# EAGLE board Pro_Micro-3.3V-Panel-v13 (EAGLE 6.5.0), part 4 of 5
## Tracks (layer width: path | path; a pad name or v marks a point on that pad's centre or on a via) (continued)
N$120 (continued)
  Top 0.203: Y14.3 36.66,84.61 C123.1 35.82,86.19 33.86,86.19 33.48,86.56 33.48,87.13 32.43,88.18 31.7,88.18 31.24,88.64 31.24,88.89 30.89,89.25 30.89,90.16 30.4,90.65 30.4,91.22 30.78,91.6 31.15,91.6 31.33,91.78
N$121
  Top 0.203: C125.2 29.17,98.65 30.01,97.82 30.71,97.82 U28.6
N$122
  Top 0.203: X14.D-1 34.69,108.47 34.92,108.23 36.79,108.23 37,108.43 R84.2
N$123
  Top 0.203: X14.D+1 34.04,108.25 34.44,107.85 35.94,107.85 36.78,107 R83.2
N$124
  Top 0.203: F14.2 32.64,106.42 32.89,106.67 D42.2 31.98,107.99 31.98,109.12 31.75,109.35 31.5,109.35 29.84,111 27.94,111 27.43,111.51 27.05,111.51 26.83,111.73 SJ14.1
N$125
  Top 0.203: R82.2 D41.C
N$126
  Top 0.203: R81.2 D40.C
N$127
  Top 0.203: R85.1 47.75,106.92 LED15.A
N$128
  Top 0.203: Y15.1 50.6,81.53 51.82,82.74 51.82,84.8 C133.1 51.27,86.97 50.48,87.76 49.79,87.76 49.12,88.42 49.12,88.66 48.76,89.03 48.76,90.02 48.28,90.5 48.28,91.42 | 49.27,92.13 49.14,92 48.87,92 48.28,91.42 | 48.28,91.42
N$129
  Top 0.203: Y15.3 54.95,84.61 C132.1 54.11,86.19 52.14,86.19 51.77,86.56 51.77,87.13 50.72,88.18 49.98,88.18 49.53,88.64 49.53,88.89 49.17,89.25 49.17,90.16 48.69,90.65 48.69,91.22 49.06,91.6 49.44,91.6 49.62,91.78
N$130
  Top 0.203: C134.2 47.46,98.65 48.3,97.82 48.99,97.82 U30.6
N$131
  Top 0.203: X15.D-1 52.97,108.47 53.21,108.23 55.08,108.23 55.28,108.43 R90.2
N$132
  Top 0.203: X15.D+1 52.32,108.25 52.73,107.85 54.23,107.85 55.07,107 R89.2
N$133
  Top 0.203: F15.2 50.92,106.42 51.17,106.67 D45.2 50.27,107.99 50.27,109.12 50.04,109.35 49.78,109.35 48.13,111 46.23,111 45.72,111.51 45.34,111.51 45.12,111.73 SJ15.1
N$134
  Top 0.203: R88.2 D44.C
N$135
  Top 0.203: R87.2 D43.C
N$136
  Top 0.203: R91.1 66.04,106.92 LED16.A
N$137
  Top 0.203: Y16.1 68.89,81.53 70.1,82.74 70.1,84.8 C142.1 69.56,86.97 68.77,87.76 68.08,87.76 67.41,88.42 67.41,88.66 67.04,89.03 67.04,90.02 66.57,90.5 66.57,91.42 | 67.56,92.13 67.43,92 67.16,92 66.57,91.42 | 66.57,91.42
N$138
  Top 0.203: Y16.3 73.24,84.61 C141.1 72.4,86.19 70.43,86.19 70.06,86.56 70.06,87.13 69.01,88.18 68.27,88.18 67.82,88.64 67.82,88.89 67.46,89.25 67.46,90.16 66.97,90.65 66.97,91.22 67.35,91.6 67.73,91.6 67.9,91.78
N$139
  Top 0.203: C143.2 65.75,98.65 66.58,97.82 67.28,97.82 U32.6
N$140
  Top 0.203: X16.D-1 71.26,108.47 71.5,108.23 73.37,108.23 73.57,108.43 R96.2
N$141
  Top 0.203: X16.D+1 70.61,108.25 71.02,107.85 72.52,107.85 73.36,107 R95.2
N$142
  Top 0.203: F16.2 69.21,106.42 69.46,106.67 D48.2 68.56,107.99 68.56,109.12 68.33,109.35 68.07,109.35 66.42,111 64.52,111 64.01,111.51 63.63,111.51 63.4,111.73 SJ16.1
N$143
  Top 0.203: R94.2 D47.C
N$144
  Top 0.203: R93.2 D46.C
N$145
  Top 0.203: R97.1 84.33,106.92 LED17.A
N$146
  Top 0.203: Y17.1 87.18,81.53 88.39,82.74 88.39,84.8 C151.1 87.84,86.97 87.06,87.76 86.36,87.76 85.7,88.42 85.7,88.66 85.33,89.03 85.33,90.02 84.86,90.5 84.86,91.42 | 85.84,92.13 85.72,92 85.45,92 84.86,91.42 | 84.86,91.42
N$147
  Top 0.203: Y17.3 91.53,84.61 C150.1 90.69,86.19 88.72,86.19 88.35,86.56 88.35,87.13 87.3,88.18 86.56,88.18 86.11,88.64 86.11,88.89 85.75,89.25 85.75,90.16 85.26,90.65 85.26,91.22 85.64,91.6 86.02,91.6 86.19,91.78
N$148
  Top 0.203: C152.2 84.04,98.65 84.87,97.82 85.57,97.82 U34.6
N$149
  Top 0.203: X17.D-1 89.55,108.47 89.79,108.23 91.66,108.23 91.86,108.43 R102.2
N$150
  Top 0.203: X17.D+1 88.9,108.25 89.31,107.85 90.81,107.85 91.65,107 R101.2
N$151
  Top 0.203: F17.2 87.5,106.42 87.75,106.67 D51.2 86.84,107.99 86.84,109.12 86.61,109.35 86.36,109.35 84.71,111 82.8,111 82.3,111.51 81.92,111.51 81.69,111.73 SJ17.1
N$152
  Top 0.203: R100.2 D50.C
N$153
  Top 0.203: R99.2 D49.C
N$154
  Top 0.203: R103.1 102.61,106.92 LED18.A
N$155
  Top 0.203: Y18.1 105.47,81.53 106.68,82.74 106.68,84.8 C160.1 106.13,86.97 105.35,87.76 104.65,87.76 103.99,88.42 103.99,88.66 103.62,89.03 103.62,90.02 103.15,90.5 103.15,91.42 | 104.13,92.13 104.01,92 103.73,92 103.15,91.42 | 103.15,91.42
N$156
  Top 0.203: Y18.3 109.82,84.61 C159.1 108.97,86.19 107.01,86.19 106.63,86.56 106.63,87.13 105.58,88.18 104.85,88.18 104.39,88.64 104.39,88.89 104.04,89.25 104.04,90.16 103.55,90.65 103.55,91.22 103.93,91.6 104.3,91.6 104.48,91.78
N$157
  Top 0.203: C161.2 102.32,98.65 103.16,97.82 103.86,97.82 U36.6
N$158
  Top 0.203: X18.D-1 107.84,108.47 108.08,108.23 109.94,108.23 110.15,108.43 R108.2
N$159
  Top 0.203: X18.D+1 107.19,108.25 107.59,107.85 109.09,107.85 109.94,107 R107.2
N$160
  Top 0.203: F18.2 105.79,106.42 106.04,106.67 D54.2 105.13,107.99 105.13,109.12 104.9,109.35 104.65,109.35 103,111 101.09,111 100.58,111.51 100.2,111.51 99.98,111.73 SJ18.1
N$161
  Top 0.203: R106.2 D53.C
N$162
  Top 0.203: R105.2 D52.C
RAW  (via drill 0.25)
  Top 0.203: 16.36,29.72 16.36,28.07 16.63,27.8 17.26,27.8 U2.1 | D2.1 16.23,33.43 | 16.23,33.43 15.19,34.47 v14.8,34.47 | C19.A 19.18,29.66 U2.3 17.24,29.72 16.36,29.72 | 16.36,29.72 16.36,30.59 16.22,30.74 16.22,33.42 16.23,33.43
  Bottom 0.203: JP6.1 23.37,36.58 21.34,38.61 16,38.61 14.8,37.4 v14.8,34.47
RAW1  (via drill 0.25)
  Top 0.203: 34.65,29.72 34.65,28.07 34.92,27.8 35.54,27.8 U1.1 | D6.1 34.52,33.43 | 34.52,33.43 33.48,34.47 v33.08,34.47 | C12.A 37.47,29.66 U1.3 35.53,29.72 34.65,29.72 | 34.65,29.72 34.65,30.59 34.51,30.74 34.51,33.42 34.52,33.43
  Bottom 0.203: JP3.1 41.66,36.58 39.62,38.61 34.29,38.61 33.08,37.4 v33.08,34.47
RAW2  (via drill 0.25)
  Top 0.203: 52.94,29.72 52.94,28.07 53.21,27.8 53.83,27.8 U5.1 | D9.1 52.81,33.43 | 52.81,33.43 51.77,34.47 v51.37,34.47 | C23.A 55.76,29.66 U5.3 53.81,29.72 52.94,29.72 | 52.94,29.72 52.94,30.59 52.8,30.74 52.8,33.42 52.81,33.43
  Bottom 0.203: JP9.1 59.94,36.58 57.91,38.61 52.58,38.61 51.37,37.4 v51.37,34.47
RAW3  (via drill 0.25)
  Top 0.203: 71.23,29.72 71.23,28.07 71.5,27.8 72.12,27.8 U7.1 | D12.1 71.09,33.43 | 71.09,33.43 70.05,34.47 v69.66,34.47 | C32.A 74.05,29.66 U7.3 72.1,29.72 71.23,29.72 | 71.23,29.72 71.23,30.59 71.08,30.74 71.08,33.42 71.09,33.43
  Bottom 0.203: JP13.1 78.23,36.58 76.2,38.61 70.87,38.61 69.66,37.4 v69.66,34.47
RAW4  (via drill 0.25)
  Top 0.203: 89.52,29.72 89.52,28.07 89.79,27.8 90.41,27.8 U9.1 | D15.1 89.38,33.43 | 89.38,33.43 88.34,34.47 v87.95,34.47 | C41.A 92.33,29.66 U9.3 90.39,29.72 89.52,29.72 | 89.52,29.72 89.52,30.59 89.37,30.74 89.37,33.42 89.38,33.43
  Bottom 0.203: JP17.1 96.52,36.58 94.49,38.61 89.15,38.61 87.95,37.4 v87.95,34.47
RAW5  (via drill 0.25)
  Top 0.203: 107.81,29.72 107.81,28.07 108.07,27.8 108.7,27.8 U11.1 | D18.1 107.67,33.43 | 107.67,33.43 106.63,34.47 v106.24,34.47 | C50.A 110.62,29.66 U11.3 108.68,29.72 107.81,29.72 | 107.81,29.72 107.81,30.59 107.66,30.74 107.66,33.42 107.67,33.43
  Bottom 0.203: JP21.1 114.81,36.58 112.78,38.61 107.44,38.61 106.24,37.4 v106.24,34.47
RAW6  (via drill 0.25)
  Top 0.203: 16.36,66.55 16.36,64.9 16.63,64.63 17.26,64.63 U13.1 | D21.1 16.23,70.26 | 16.23,70.26 15.19,71.3 v14.8,71.3 | C59.A 19.18,66.49 U13.3 17.24,66.55 16.36,66.55 | 16.36,66.55 16.36,67.42 16.22,67.57 16.22,70.25 16.23,70.26
  Bottom 0.203: JP25.1 23.37,73.41 21.34,75.44 16,75.44 14.8,74.23 v14.8,71.3
RAW7  (via drill 0.25)
  Top 0.203: 34.65,66.55 34.65,64.9 34.92,64.63 35.54,64.63 U15.1 | D24.1 34.52,70.26 | 34.52,70.26 33.48,71.3 v33.08,71.3 | C68.A 37.47,66.49 U15.3 35.53,66.55 34.65,66.55 | 34.65,66.55 34.65,67.42 34.51,67.57 34.51,70.25 34.52,70.26
  Bottom 0.203: JP29.1 41.66,73.41 39.62,75.44 34.29,75.44 33.08,74.23 v33.08,71.3
RAW8  (via drill 0.25)
  Top 0.203: 52.94,66.55 52.94,64.9 53.21,64.63 53.83,64.63 U17.1 | D27.1 52.81,70.26 | 52.81,70.26 51.77,71.3 v51.37,71.3 | C77.A 55.76,66.49 U17.3 53.81,66.55 52.94,66.55 | 52.94,66.55 52.94,67.42 52.8,67.57 52.8,70.25 52.81,70.26
  Bottom 0.203: JP33.1 59.94,73.41 57.91,75.44 52.58,75.44 51.37,74.23 v51.37,71.3
RAW9  (via drill 0.25)
  Top 0.203: 71.23,66.55 71.23,64.9 71.5,64.63 72.12,64.63 U19.1 | D30.1 71.09,70.26 | 71.09,70.26 70.05,71.3 v69.66,71.3 | C86.A 74.05,66.49 U19.3 72.1,66.55 71.23,66.55 | 71.23,66.55 71.23,67.42 71.08,67.57 71.08,70.25 71.09,70.26
  Bottom 0.203: JP37.1 78.23,73.41 76.2,75.44 70.87,75.44 69.66,74.23 v69.66,71.3
RAW10  (via drill 0.25)
  Top 0.203: 89.52,66.55 89.52,64.9 89.79,64.63 90.41,64.63 U21.1 | D33.1 89.38,70.26 | 89.38,70.26 88.34,71.3 v87.95,71.3 | C95.A 92.33,66.49 U21.3 90.39,66.55 89.52,66.55 | 89.52,66.55 89.52,67.42 89.37,67.57 89.37,70.25 89.38,70.26
  Bottom 0.203: JP41.1 96.52,73.41 94.49,75.44 89.15,75.44 87.95,74.23 v87.95,71.3
RAW11  (via drill 0.25)
  Top 0.203: 107.81,66.55 107.81,64.9 108.07,64.63 108.7,64.63 U23.1 | D36.1 107.67,70.26 | 107.67,70.26 106.63,71.3 v106.24,71.3 | C104.A 110.62,66.49 U23.3 108.68,66.55 107.81,66.55 | 107.81,66.55 107.81,67.42 107.66,67.57 107.66,70.25 107.67,70.26
  Bottom 0.203: JP45.1 114.81,73.41 112.78,75.44 107.44,75.44 106.24,74.23 v106.24,71.3
RAW12  (via drill 0.25)
  Top 0.203: 16.36,103.38 16.36,101.73 16.63,101.46 17.26,101.46 U25.1 | D39.1 16.23,107.09 | 16.23,107.09 15.19,108.13 v14.8,108.13 | C113.A 19.18,103.32 U25.3 17.24,103.38 16.36,103.38 | 16.36,103.38 16.36,104.25 16.22,104.4 16.22,107.08 16.23,107.09
  Bottom 0.203: JP49.1 23.37,110.24 21.34,112.27 16,112.27 14.8,111.06 v14.8,108.13
RAW13  (via drill 0.25)
  Top 0.203: 34.65,103.38 34.65,101.73 34.92,101.46 35.54,101.46 U27.1 | D42.1 34.52,107.09 | 34.52,107.09 33.48,108.13 v33.08,108.13 | C122.A 37.47,103.32 U27.3 35.53,103.38 34.65,103.38 | 34.65,103.38 34.65,104.25 34.51,104.4 34.51,107.08 34.52,107.09
  Bottom 0.203: JP53.1 41.66,110.24 39.62,112.27 34.29,112.27 33.08,111.06 v33.08,108.13
RAW14  (via drill 0.25)
  Top 0.203: 52.94,103.38 52.94,101.73 53.21,101.46 53.83,101.46 U29.1 | D45.1 52.81,107.09 | 52.81,107.09 51.77,108.13 v51.37,108.13 | C131.A 55.76,103.32 U29.3 53.81,103.38 52.94,103.38 | 52.94,103.38 52.94,104.25 52.8,104.4 52.8,107.08 52.81,107.09
  Bottom 0.203: JP57.1 59.94,110.24 57.91,112.27 52.58,112.27 51.37,111.06 v51.37,108.13
RAW15  (via drill 0.25)
  Top 0.203: 71.23,103.38 71.23,101.73 71.5,101.46 72.12,101.46 U31.1 | D48.1 71.09,107.09 | 71.09,107.09 70.05,108.13 v69.66,108.13 | C140.A 74.05,103.32 U31.3 72.1,103.38 71.23,103.38 | 71.23,103.38 71.23,104.25 71.08,104.4 71.08,107.08 71.09,107.09
  Bottom 0.203: JP61.1 78.23,110.24 76.2,112.27 70.87,112.27 69.66,111.06 v69.66,108.13
RAW16  (via drill 0.25)
  Top 0.203: 89.52,103.38 89.52,101.73 89.79,101.46 90.41,101.46 U33.1 | D51.1 89.38,107.09 | 89.38,107.09 88.34,108.13 v87.95,108.13 | C149.A 92.33,103.32 U33.3 90.39,103.38 89.52,103.38 | 89.52,103.38 89.52,104.25 89.37,104.4 89.37,107.08 89.38,107.09
  Bottom 0.203: JP65.1 96.52,110.24 94.49,112.27 89.15,112.27 87.95,111.06 v87.95,108.13
RAW17  (via drill 0.25)
  Top 0.203: 107.81,103.38 107.81,101.73 108.07,101.46 108.7,101.46 U35.1 | D54.1 107.67,107.09 | 107.67,107.09 106.63,108.13 v106.24,108.13 | C158.A 110.62,103.32 U35.3 108.68,103.38 107.81,103.38 | 107.81,103.38 107.81,104.25 107.66,104.4 107.66,107.08 107.67,107.09
  Bottom 0.203: JP69.1 114.81,110.24 112.78,112.27 107.44,112.27 106.24,111.06 v106.24,108.13
RESET  (via drill 0.25)
  Top 0.203: 11.65,19.52 11.57,19.44 11.57,19.43 11.42,19.28 11.2,19.28 10.69,19.79 10.69,20.34 10.92,20.57 10.92,21.08 9.4,22.61 9.4,31.47 8.84,32.03 8.84,32.45 9.4,33.01 9.4,35.18 v10.29,36.07 11.09,35.27 R2.1
  Bottom 0.203: JP6.3 22.1,32.26 22.1,34.04 22.48,34.42 22.48,35.18 22.1,35.56 22.1,37.08 21.01,38.18 18.16,38.18 16.79,36.8 16.79,34.29 15.8,33.3 13.06,33.3 v10.29,36.07
RESET1  (via drill 0.25)
  Top 0.203: 29.93,19.52 29.86,19.44 29.86,19.43 29.71,19.28 29.49,19.28 28.98,19.79 28.98,20.34 29.21,20.57 29.21,21.08 27.69,22.61 27.69,31.47 27.12,32.03 27.12,32.45 27.69,33.01 27.69,35.18 v28.57,36.07 29.38,35.27 R3.1
  Bottom 0.203: JP3.3 40.39,32.26 40.39,34.04 40.77,34.42 40.77,35.18 40.39,35.56 40.39,37.08 39.29,38.18 36.45,38.18 35.08,36.8 35.08,34.29 34.09,33.3 31.34,33.3 v28.57,36.07
RESET2  (via drill 0.25)
  Top 0.203: 48.22,19.52 48.15,19.44 48.15,19.43 48,19.28 47.78,19.28 47.27,19.79 47.27,20.34 47.5,20.57 47.5,21.08 45.97,22.61 45.97,31.47 45.41,32.03 45.41,32.45 45.97,33.01 45.97,35.18 v46.86,36.07 47.66,35.27 R14.1
  Bottom 0.203: JP9.3 58.67,32.26 58.67,34.04 59.05,34.42 59.05,35.18 58.67,35.56 58.67,37.08 57.58,38.18 54.74,38.18 53.37,36.8 53.37,34.29 52.38,33.3 49.63,33.3 v46.86,36.07
RESET3  (via drill 0.25)
  Top 0.203: 66.51,19.52 66.44,19.44 66.44,19.43 66.28,19.28 66.06,19.28 65.56,19.79 65.56,20.34 65.79,20.57 65.79,21.08 64.26,22.61 64.26,31.47 63.7,32.03 63.7,32.45 64.26,33.01 64.26,35.18 v65.15,36.07 65.95,35.27 R20.1
  Bottom 0.203: JP13.3 76.96,32.26 76.96,34.04 77.34,34.42 77.34,35.18 76.96,35.56 76.96,37.08 75.87,38.18 73.03,38.18 71.65,36.8 71.65,34.29 70.66,33.3 67.92,33.3 v65.15,36.07
RESET4  (via drill 0.25)
  Top 0.203: 84.8,19.52 84.72,19.44 84.72,19.43 84.57,19.28 84.35,19.28 83.84,19.79 83.84,20.34 84.07,20.57 84.07,21.08 82.55,22.61 82.55,31.47 81.99,32.03 81.99,32.45 82.55,33.01 82.55,35.18 v83.44,36.07 84.24,35.27 R26.1
  Bottom 0.203: JP17.3 95.25,32.26 95.25,34.04 95.63,34.42 95.63,35.18 95.25,35.56 95.25,37.08 94.16,38.18 91.31,38.18 89.94,36.8 89.94,34.29 88.95,33.3 86.21,33.3 v83.44,36.07
RESET5  (via drill 0.25)
  Top 0.203: 103.09,19.52 103.01,19.44 103.01,19.43 102.86,19.28 102.64,19.28 102.13,19.79 102.13,20.34 102.36,20.57 102.36,21.08 100.84,22.61 100.84,31.47 100.28,32.03 100.28,32.45 100.84,33.01 100.84,35.18 v101.73,36.07 102.53,35.27 R32.1
  Bottom 0.203: JP21.3 113.54,32.26 113.54,34.04 113.92,34.42 113.92,35.18 113.54,35.56 113.54,37.08 112.45,38.18 109.6,38.18 108.23,36.8 108.23,34.29 107.24,33.3 104.5,33.3 v101.73,36.07
RESET6  (via drill 0.25)
  Top 0.203: 11.65,56.34 11.57,56.27 11.57,56.26 11.42,56.11 11.2,56.11 10.69,56.62 10.69,57.17 10.92,57.4 10.92,57.91 9.4,59.44 9.4,68.3 8.84,68.86 8.84,69.28 9.4,69.84 9.4,72.01 v10.29,72.9 11.09,72.1 R38.1
  Bottom 0.203: JP25.3 22.1,69.09 22.1,70.87 22.48,71.25 22.48,72.01 22.1,72.39 22.1,73.91 21.01,75.01 18.16,75.01 16.79,73.64 16.79,71.12 15.8,70.13 13.06,70.13 v10.29,72.9
RESET7  (via drill 0.25)
  Top 0.203: 29.93,56.34 29.86,56.27 29.86,56.26 29.71,56.11 29.49,56.11 28.98,56.62 28.98,57.17 29.21,57.4 29.21,57.91 27.69,59.44 27.69,68.3 27.12,68.86 27.12,69.28 27.69,69.84 27.69,72.01 v28.57,72.9 29.38,72.1 R44.1
  Bottom 0.203: JP29.3 40.39,69.09 40.39,70.87 40.77,71.25 40.77,72.01 40.39,72.39 40.39,73.91 39.29,75.01 36.45,75.01 35.08,73.64 35.08,71.12 34.09,70.13 31.34,70.13 v28.57,72.9
RESET8  (via drill 0.25)
  Top 0.203: 48.22,56.34 48.15,56.27 48.15,56.26 48,56.11 47.78,56.11 47.27,56.62 47.27,57.17 47.5,57.4 47.5,57.91 45.97,59.44 45.97,68.3 45.41,68.86 45.41,69.28 45.97,69.84 45.97,72.01 v46.86,72.9 47.66,72.1 R50.1
  Bottom 0.203: JP33.3 58.67,69.09 58.67,70.87 59.05,71.25 59.05,72.01 58.67,72.39 58.67,73.91 57.58,75.01 54.74,75.01 53.37,73.64 53.37,71.12 52.38,70.13 49.63,70.13 v46.86,72.9
RESET9  (via drill 0.25)
  Top 0.203: 66.51,56.34 66.44,56.27 66.44,56.26 66.28,56.11 66.06,56.11 65.56,56.62 65.56,57.17 65.79,57.4 65.79,57.91 64.26,59.44 64.26,68.3 63.7,68.86 63.7,69.28 64.26,69.84 64.26,72.01 v65.15,72.9 65.95,72.1 R56.1
  Bottom 0.203: JP37.3 76.96,69.09 76.96,70.87 77.34,71.25 77.34,72.01 76.96,72.39 76.96,73.91 75.87,75.01 73.03,75.01 71.65,73.64 71.65,71.12 70.66,70.13 67.92,70.13 v65.15,72.9
RESET10  (via drill 0.25)
  Top 0.203: 84.8,56.34 84.72,56.27 84.72,56.26 84.57,56.11 84.35,56.11 83.84,56.62 83.84,57.17 84.07,57.4 84.07,57.91 82.55,59.44 82.55,68.3 81.99,68.86 81.99,69.28 82.55,69.84 82.55,72.01 v83.44,72.9 84.24,72.1 R62.1
  Bottom 0.203: JP41.3 95.25,69.09 95.25,70.87 95.63,71.25 95.63,72.01 95.25,72.39 95.25,73.91 94.16,75.01 91.31,75.01 89.94,73.64 89.94,71.12 88.95,70.13 86.21,70.13 v83.44,72.9
RESET11  (via drill 0.25)
  Top 0.203: 103.09,56.34 103.01,56.27 103.01,56.26 102.86,56.11 102.64,56.11 102.13,56.62 102.13,57.17 102.36,57.4 102.36,57.91 100.84,59.44 100.84,68.3 100.28,68.86 100.28,69.28 100.84,69.84 100.84,72.01 v101.73,72.9 102.53,72.1 R68.1
  Bottom 0.203: JP45.3 113.54,69.09 113.54,70.87 113.92,71.25 113.92,72.01 113.54,72.39 113.54,73.91 112.45,75.01 109.6,75.01 108.23,73.64 108.23,71.12 107.24,70.13 104.5,70.13 v101.73,72.9
RESET12  (via drill 0.25)
  Top 0.203: 11.65,93.17 11.57,93.1 11.57,93.09 11.42,92.94 11.2,92.94 10.69,93.45 10.69,94 10.92,94.23 10.92,94.74 9.4,96.27 9.4,105.13 8.84,105.69 8.84,106.11 9.4,106.67 9.4,108.84 v10.29,109.73 11.09,108.93 R74.1
  Bottom 0.203: JP49.3 22.1,105.92 22.1,107.7 22.48,108.08 22.48,108.84 22.1,109.22 22.1,110.74 21.01,111.84 18.16,111.84 16.79,110.47 16.79,107.95 15.8,106.96 13.06,106.96 v10.29,109.73
RESET13  (via drill 0.25)
  Top 0.203: 29.93,93.17 29.86,93.1 29.86,93.09 29.71,92.94 29.49,92.94 28.98,93.45 28.98,94 29.21,94.23 29.21,94.74 27.69,96.27 27.69,105.13 27.12,105.69 27.12,106.11 27.69,106.67 27.69,108.84 v28.57,109.73 29.38,108.93 R80.1
  Bottom 0.203: JP53.3 40.39,105.92 40.39,107.7 40.77,108.08 40.77,108.84 40.39,109.22 40.39,110.74 39.29,111.84 36.45,111.84 35.08,110.47 35.08,107.95 34.09,106.96 31.34,106.96 v28.57,109.73
RESET14  (via drill 0.25)
  Top 0.203: 48.22,93.17 48.15,93.1 48.15,93.09 48,92.94 47.78,92.94 47.27,93.45 47.27,94 47.5,94.23 47.5,94.74 45.97,96.27 45.97,105.13 45.41,105.69 45.41,106.11 45.97,106.67 45.97,108.84 v46.86,109.73 47.66,108.93 R86.1
  Bottom 0.203: JP57.3 58.67,105.92 58.67,107.7 59.05,108.08 59.05,108.84 58.67,109.22 58.67,110.74 57.58,111.84 54.74,111.84 53.37,110.47 53.37,107.95 52.38,106.96 49.63,106.96 v46.86,109.73
RESET15  (via drill 0.25)
  Top 0.203: 66.51,93.17 66.44,93.1 66.44,93.09 66.28,92.94 66.06,92.94 65.56,93.45 65.56,94 65.79,94.23 65.79,94.74 64.26,96.27 64.26,105.13 63.7,105.69 63.7,106.11 64.26,106.67 64.26,108.84 v65.15,109.73 65.95,108.93 R92.1
  Bottom 0.203: JP61.3 76.96,105.92 76.96,107.7 77.34,108.08 77.34,108.84 76.96,109.22 76.96,110.74 75.87,111.84 73.03,111.84 71.65,110.47 71.65,107.95 70.66,106.96 67.92,106.96 v65.15,109.73
RESET16  (via drill 0.25)
  Top 0.203: 84.8,93.17 84.72,93.1 84.72,93.09 84.57,92.94 84.35,92.94 83.84,93.45 83.84,94 84.07,94.23 84.07,94.74 82.55,96.27 82.55,105.13 81.99,105.69 81.99,106.11 82.55,106.67 82.55,108.84 v83.44,109.73 84.24,108.93 R98.1
  Bottom 0.203: JP65.3 95.25,105.92 95.25,107.7 95.63,108.08 95.63,108.84 95.25,109.22 95.25,110.74 94.16,111.84 91.31,111.84 89.94,110.47 89.94,107.95 88.95,106.96 86.21,106.96 v83.44,109.73
RESET17  (via drill 0.25)
  Top 0.203: 103.09,93.17 103.01,93.1 103.01,93.09 102.86,92.94 102.64,92.94 102.13,93.45 102.13,94 102.36,94.23 102.36,94.74 100.84,96.27 100.84,105.13 100.28,105.69 100.28,106.11 100.84,106.67 100.84,108.84 v101.73,109.73 102.53,108.93 R104.1
  Bottom 0.203: JP69.3 113.54,105.92 113.54,107.7 113.92,108.08 113.92,108.84 113.54,109.22 113.54,110.74 112.45,111.84 109.6,111.84 108.23,110.47 108.23,107.95 107.24,106.96 104.5,106.96 v101.73,109.73
RXI  (via drill 0.25)
  Top 0.203: 14.09,17.07 14,16.98 13.99,16.98 13.99,15.72 v13.61,15.34
  Bottom 0.203: JP7.11 10.09,33.53 12.13,31.49 12.13,28.09 11.22,27.18 10.57,27.18 10.57,27.16 10.18,26.77 10.18,24.73 10.38,24.53 | v13.61,15.34 14.89,16.61 14.89,18.46 12.12,21.23 12.12,23.68 11.26,24.53 10.38,24.53 | 10.38,24.53 10.37,24.53
RXI1  (via drill 0.25)
  Top 0.203: 32.37,17.07 32.28,16.98 32.28,15.72 v31.9,15.34
  Bottom 0.203: JP4.11 28.38,33.53 30.42,31.49 30.42,28.09 29.51,27.18 28.86,27.18 28.86,27.16 28.47,26.77 28.47,24.73 28.66,24.53 | v31.9,15.34 33.17,16.61 33.17,18.46 30.4,21.23 30.4,23.68 29.55,24.53 28.66,24.53 | 28.66,24.53 28.65,24.53
RXI2  (via drill 0.25)
  Top 0.203: 50.66,17.07 50.57,16.98 50.57,15.72 v50.19,15.34
  Bottom 0.203: JP10.11 46.67,33.53 48.71,31.49 48.71,28.09 47.8,27.18 47.15,27.18 47.15,27.16 46.75,26.77 46.75,24.73 46.95,24.53 | v50.19,15.34 51.46,16.61 51.46,18.46 48.69,21.23 48.69,23.68 47.84,24.53 46.95,24.53 | 46.95,24.53 46.94,24.53
RXI3  (via drill 0.25)
  Top 0.203: 68.95,17.07 68.86,16.98 68.86,15.72 v68.48,15.34
  Bottom 0.203: JP14.11 64.95,33.53 67,31.49 67,28.09 66.08,27.18 65.44,27.18 65.44,27.16 65.04,26.77 65.04,24.73 65.24,24.53 | v68.48,15.34 69.75,16.61 69.75,18.46 66.98,21.23 66.98,23.68 66.12,24.53 65.24,24.53 | 65.24,24.53 65.23,24.53
RXI4  (via drill 0.25)
  Top 0.203: 87.24,17.07 87.15,16.98 87.15,15.72 v86.76,15.34
  Bottom 0.203: JP18.11 83.24,33.53 85.28,31.49 85.28,28.09 84.37,27.18 83.73,27.18 83.73,27.16 83.33,26.77 83.33,24.73 83.53,24.53 | v86.76,15.34 88.04,16.61 88.04,18.46 85.27,21.23 85.27,23.68 84.41,24.53 83.53,24.53 | 83.53,24.53 83.52,24.53
RXI5  (via drill 0.25)
  Top 0.203: 105.53,17.07 105.44,16.98 105.44,15.72 v105.05,15.34
  Bottom 0.203: JP22.11 101.53,33.53 103.57,31.49 103.57,28.09 102.66,27.18 102.01,27.18 102.01,27.16 101.62,26.77 101.62,24.73 101.82,24.53 | v105.05,15.34 106.33,16.61 106.33,18.46 103.56,21.23 103.56,23.68 102.7,24.53 101.82,24.53 | 101.82,24.53 101.81,24.53
RXI6  (via drill 0.25)
  Top 0.203: 14.09,53.9 14,53.81 13.99,53.81 13.99,52.55 v13.61,52.17
  Bottom 0.203: JP26.11 10.09,70.36 12.13,68.32 12.13,64.92 11.22,64 10.57,64 10.57,63.99 10.18,63.6 10.18,61.56 10.38,61.36 | v13.61,52.17 14.89,53.44 14.89,55.29 12.12,58.06 12.12,60.51 11.26,61.36 10.38,61.36 | 10.38,61.36 10.37,61.36
RXI7  (via drill 0.25)
  Top 0.203: 32.37,53.9 32.28,53.81 32.28,52.55 v31.9,52.17
  Bottom 0.203: JP30.11 28.38,70.36 30.42,68.32 30.42,64.92 29.51,64 28.86,64 28.86,63.99 28.47,63.6 28.47,61.56 28.66,61.36 | v31.9,52.17 33.17,53.44 33.17,55.29 30.4,58.06 30.4,60.51 29.55,61.36 28.66,61.36 | 28.66,61.36 28.65,61.36
RXI8  (via drill 0.25)
  Top 0.203: 50.66,53.9 50.57,53.81 50.57,52.55 v50.19,52.17
  Bottom 0.203: JP34.11 46.67,70.36 48.71,68.32 48.71,64.92 47.8,64 47.15,64 47.15,63.99 46.75,63.6 46.75,61.56 46.95,61.36 | v50.19,52.17 51.46,53.44 51.46,55.29 48.69,58.06 48.69,60.51 47.84,61.36 46.95,61.36 | 46.95,61.36 46.94,61.36
RXI9  (via drill 0.25)
  Top 0.203: 68.95,53.9 68.86,53.81 68.86,52.55 v68.48,52.17
  Bottom 0.203: JP38.11 64.95,70.36 67,68.32 67,64.92 66.08,64 65.44,64 65.44,63.99 65.04,63.6 65.04,61.56 65.24,61.36 | v68.48,52.17 69.75,53.44 69.75,55.29 66.98,58.06 66.98,60.51 66.12,61.36 65.24,61.36 | 65.24,61.36 65.23,61.36
RXI10  (via drill 0.25)
  Top 0.203: 87.24,53.9 87.15,53.81 87.15,52.55 v86.76,52.17
  Bottom 0.203: JP42.11 83.24,70.36 85.28,68.32 85.28,64.92 84.37,64 83.73,64 83.73,63.99 83.33,63.6 83.33,61.56 83.53,61.36 | v86.76,52.17 88.04,53.44 88.04,55.29 85.27,58.06 85.27,60.51 84.41,61.36 83.53,61.36 | 83.53,61.36 83.52,61.36
RXI11  (via drill 0.25)
  Top 0.203: 105.53,53.9 105.44,53.81 105.44,52.55 v105.05,52.17
  Bottom 0.203: JP46.11 101.53,70.36 103.57,68.32 103.57,64.92 102.66,64 102.01,64 102.01,63.99 101.62,63.6 101.62,61.56 101.82,61.36 | v105.05,52.17 106.33,53.44 106.33,55.29 103.56,58.06 103.56,60.51 102.7,61.36 101.82,61.36 | 101.82,61.36 101.81,61.36
RXI12  (via drill 0.25)
  Top 0.203: 14.09,90.73 14,90.64 13.99,90.64 13.99,89.38 v13.61,89
  Bottom 0.203: JP50.11 10.09,107.19 12.13,105.15 12.13,101.75 11.22,100.83 10.57,100.83 10.18,100.43 10.18,98.39 10.38,98.19 | v13.61,89 14.89,90.27 14.89,92.12 12.12,94.89 12.12,97.33 11.26,98.19 10.38,98.19 | 10.38,98.19 10.37,98.19
RXI13  (via drill 0.25)
  Top 0.203: 32.37,90.73 32.28,90.64 32.28,89.38 v31.9,89
  Bottom 0.203: JP54.11 28.38,107.19 30.42,105.15 30.42,101.75 29.51,100.83 28.86,100.83 28.47,100.43 28.47,98.39 28.66,98.19 | v31.9,89 33.17,90.27 33.17,92.12 30.4,94.89 30.4,97.33 29.55,98.19 28.66,98.19 | 28.66,98.19 28.65,98.19
RXI14  (via drill 0.25)
  Top 0.203: 50.66,90.73 50.57,90.64 50.57,89.38 v50.19,89
  Bottom 0.203: JP58.11 46.67,107.19 48.71,105.15 48.71,101.75 47.8,100.83 47.15,100.83 46.75,100.43 46.75,98.39 46.95,98.19 | v50.19,89 51.46,90.27 51.46,92.12 48.69,94.89 48.69,97.33 47.84,98.19 46.95,98.19 | 46.95,98.19 46.94,98.19
RXI15  (via drill 0.25)
  Top 0.203: 68.95,90.73 68.86,90.64 68.86,89.38 v68.48,89
  Bottom 0.203: JP62.11 64.95,107.19 67,105.15 67,101.75 66.08,100.83 65.44,100.83 65.04,100.43 65.04,98.39 65.24,98.19 | v68.48,89 69.75,90.27 69.75,92.12 66.98,94.89 66.98,97.33 66.12,98.19 65.24,98.19 | 65.24,98.19 65.23,98.19
RXI16  (via drill 0.25)
  Top 0.203: 87.24,90.73 87.15,90.64 87.15,89.38 v86.76,89
  Bottom 0.203: JP66.11 83.24,107.19 85.28,105.15 85.28,101.75 84.37,100.83 83.73,100.83 83.33,100.43 83.33,98.39 83.53,98.19 | v86.76,89 88.04,90.27 88.04,92.12 85.27,94.89 85.27,97.33 84.41,98.19 83.53,98.19 | 83.53,98.19 83.52,98.19
RXI17  (via drill 0.25)
  Top 0.203: 105.53,90.73 105.44,90.64 105.44,89.38 v105.05,89
  Bottom 0.203: JP70.11 101.53,107.19 103.57,105.15 103.57,101.75 102.66,100.83 102.01,100.83 101.62,100.43 101.62,98.39 101.82,98.19 | v105.05,89 106.33,90.27 106.33,92.12 103.56,94.89 103.56,97.33 102.7,98.19 101.82,98.19 | 101.82,98.19 101.81,98.19
SCK  (via drill 0.25)
  Top 0.203: v17.02,22.1 16.76,21.84 12.64,21.84 | 12.61,21.84 12.64,21.84 | U3.9 12.64,21.84
  Bottom 0.203: JP6.9 22.1,17.02 22.1,20.57 21.59,21.08 20.95,21.08 20.45,21.59 17.78,21.59 17.27,22.1 v17.02,22.1
SCK1  (via drill 0.25)
  Top 0.203: v35.31,22.1 35.05,21.84 30.93,21.84 | 30.9,21.84 30.93,21.84 | U4.9 30.93,21.84
  Bottom 0.203: JP3.9 40.39,17.02 40.39,20.57 39.88,21.08 39.24,21.08 38.73,21.59 36.07,21.59 35.56,22.1 v35.31,22.1
SCK2  (via drill 0.25)
  Top 0.203: v53.59,22.1 53.34,21.84 49.22,21.84 | 49.19,21.84 49.22,21.84 | U6.9 49.22,21.84
  Bottom 0.203: JP9.9 58.67,17.02 58.67,20.57 58.17,21.08 57.53,21.08 57.02,21.59 54.36,21.59 53.85,22.1 v53.59,22.1
SCK3  (via drill 0.25)
  Top 0.203: v71.88,22.1 71.63,21.84 67.5,21.84 | 67.47,21.84 67.5,21.84 | U8.9 67.5,21.84
  Bottom 0.203: JP13.9 76.96,17.02 76.96,20.57 76.45,21.08 75.82,21.08 75.31,21.59 72.64,21.59 72.14,22.1 v71.88,22.1
SCK4  (via drill 0.25)
  Top 0.203: v90.17,22.1 89.92,21.84 85.79,21.84 | 85.76,21.84 85.79,21.84 | U10.9 85.79,21.84
  Bottom 0.203: JP17.9 95.25,17.02 95.25,20.57 94.74,21.08 94.11,21.08 93.6,21.59 90.93,21.59 90.42,22.1 v90.17,22.1
SCK5  (via drill 0.25)
  Top 0.203: v108.46,22.1 108.2,21.84 104.08,21.84 | 104.05,21.84 104.08,21.84 | U12.9 104.08,21.84
  Bottom 0.203: JP21.9 113.54,17.02 113.54,20.57 113.03,21.08 112.39,21.08 111.89,21.59 109.22,21.59 108.71,22.1 v108.46,22.1
SCK6  (via drill 0.25)
  Top 0.203: v17.02,58.93 16.76,58.67 12.64,58.67 | 12.61,58.67 12.64,58.67 | U14.9 12.64,58.67
  Bottom 0.203: JP25.9 22.1,53.85 22.1,57.4 21.59,57.91 20.95,57.91 20.45,58.42 17.78,58.42 17.27,58.93 v17.02,58.93
SCK7  (via drill 0.25)
  Top 0.203: v35.31,58.93 35.05,58.67 30.93,58.67 | 30.9,58.67 30.93,58.67 | U16.9 30.93,58.67
  Bottom 0.203: JP29.9 40.39,53.85 40.39,57.4 39.88,57.91 39.24,57.91 38.73,58.42 36.07,58.42 35.56,58.93 v35.31,58.93
SCK8  (via drill 0.25)
  Top 0.203: v53.59,58.93 53.34,58.67 49.22,58.67 | 49.19,58.67 49.22,58.67 | U18.9 49.22,58.67
  Bottom 0.203: JP33.9 58.67,53.85 58.67,57.4 58.17,57.91 57.53,57.91 57.02,58.42 54.36,58.42 53.85,58.93 v53.59,58.93
SCK9  (via drill 0.25)
  Top 0.203: v71.88,58.93 71.63,58.67 67.5,58.67 | 67.47,58.67 67.5,58.67 | U20.9 67.5,58.67
  Bottom 0.203: JP37.9 76.96,53.85 76.96,57.4 76.45,57.91 75.82,57.91 75.31,58.42 72.64,58.42 72.14,58.93 v71.88,58.93
SCK10  (via drill 0.25)
  Top 0.203: v90.17,58.93 89.92,58.67 85.79,58.67 | 85.76,58.67 85.79,58.67 | U22.9 85.79,58.67
  Bottom 0.203: JP41.9 95.25,53.85 95.25,57.4 94.74,57.91 94.11,57.91 93.6,58.42 90.93,58.42 90.42,58.93 v90.17,58.93
SCK11  (via drill 0.25)
  Top 0.203: v108.46,58.93 108.2,58.67 104.08,58.67 | 104.05,58.67 104.08,58.67 | U24.9 104.08,58.67
  Bottom 0.203: JP45.9 113.54,53.85 113.54,57.4 113.03,57.91 112.39,57.91 111.89,58.42 109.22,58.42 108.71,58.93 v108.46,58.93
SCK12  (via drill 0.25)
  Top 0.203: v17.02,95.76 16.76,95.5 12.64,95.5 | 12.61,95.5 12.64,95.5 | U26.9 12.64,95.5
  Bottom 0.203: JP49.9 22.1,90.68 22.1,94.23 21.59,94.74 20.95,94.74 20.45,95.25 17.78,95.25 17.27,95.76 v17.02,95.76
SCK13  (via drill 0.25)
  Top 0.203: v35.31,95.76 35.05,95.5 30.93,95.5 | 30.9,95.5 30.93,95.5 | U28.9 30.93,95.5
  Bottom 0.203: JP53.9 40.39,90.68 40.39,94.23 39.88,94.74 39.24,94.74 38.73,95.25 36.07,95.25 35.56,95.76 v35.31,95.76
SCK14  (via drill 0.25)
  Top 0.203: v53.59,95.76 53.34,95.5 49.22,95.5 | 49.19,95.5 49.22,95.5 | U30.9 49.22,95.5
  Bottom 0.203: JP57.9 58.67,90.68 58.67,94.23 58.17,94.74 57.53,94.74 57.02,95.25 54.36,95.25 53.85,95.76 v53.59,95.76
SCK15  (via drill 0.25)
  Top 0.203: v71.88,95.76 71.63,95.5 67.5,95.5 | 67.47,95.5 67.5,95.5 | U32.9 67.5,95.5
  Bottom 0.203: JP61.9 76.96,90.68 76.96,94.23 76.45,94.74 75.82,94.74 75.31,95.25 72.64,95.25 72.14,95.76 v71.88,95.76
SCK16  (via drill 0.25)
  Top 0.203: v90.17,95.76 89.92,95.5 85.79,95.5 | 85.76,95.5 85.79,95.5 | U34.9 85.79,95.5
  Bottom 0.203: JP65.9 95.25,90.68 95.25,94.23 94.74,94.74 94.11,94.74 93.6,95.25 90.93,95.25 90.42,95.76 v90.17,95.76
SCK17  (via drill 0.25)
  Top 0.203: v108.46,95.76 108.2,95.5 104.08,95.5 | 104.05,95.5 104.08,95.5 | U36.9 104.08,95.5
  Bottom 0.203: JP69.9 113.54,90.68 113.54,94.23 113.03,94.74 112.39,94.74 111.89,95.25 109.22,95.25 108.71,95.76 v108.46,95.76
TXLED
  Top 0.203: 14.78,16.38 14.79,16.38 14.8,16.38 14.8,15.91 15.29,15.41 15.29,14.2 15.61,13.89 15.61,13.11 15.77,12.95 17.76,12.95 18.12,12.58 18.99,12.58 19.28,12.29 19.28,8.57 R6.1
TXLED1
  Top 0.203: 33.07,16.38 33.08,16.38 33.08,15.91 33.58,15.41 33.58,14.2 33.9,13.89 33.9,13.11 34.06,12.95 36.05,12.95 36.41,12.58 37.28,12.58 37.57,12.29 37.57,8.57 R8.1
TXLED2
  Top 0.203: 51.36,16.38 51.37,16.38 51.37,15.91 51.87,15.41 51.87,14.2 52.18,13.89 52.18,13.11 52.34,12.95 54.33,12.95 54.7,12.58 55.57,12.58 55.85,12.29 55.85,8.57 R15.1
TXLED3
  Top 0.203: 69.65,16.38 69.66,16.38 69.66,15.91 70.16,15.41 70.16,14.2 70.47,13.89 70.47,13.11 70.63,12.95 72.62,12.95 72.99,12.58 73.86,12.58 74.14,12.29 74.14,8.57 R21.1
TXLED4
  Top 0.203: 87.94,16.38 87.95,16.38 87.95,15.91 88.44,15.41 88.44,14.2 88.76,13.89 88.76,13.11 88.92,12.95 90.91,12.95 91.28,12.58 92.14,12.58 92.43,12.29 92.43,8.57 R27.1
TXLED5
  Top 0.203: 106.22,16.38 106.23,16.38 106.24,16.38 106.24,15.91 106.73,15.41 106.73,14.2 107.05,13.89 107.05,13.11 107.21,12.95 109.2,12.95 109.56,12.58 110.43,12.58 110.72,12.29 110.72,8.57 R33.1
TXLED6
  Top 0.203: 14.78,53.21 14.79,53.21 14.8,53.21 14.8,52.74 15.29,52.24 15.29,51.03 15.61,50.72 15.61,49.94 15.77,49.78 17.76,49.78 18.12,49.41 18.99,49.41 19.28,49.12 19.28,45.4 R39.1
TXLED7
  Top 0.203: 33.07,53.21 33.08,53.21 33.08,52.74 33.58,52.24 33.58,51.03 33.9,50.72 33.9,49.94 34.06,49.78 36.05,49.78 36.41,49.41 37.28,49.41 37.57,49.12 37.57,45.4 R45.1
TXLED8
  Top 0.203: 51.36,53.21 51.37,53.21 51.37,52.74 51.87,52.24 51.87,51.03 52.18,50.72 52.18,49.94 52.34,49.78 54.33,49.78 54.7,49.41 55.57,49.41 55.85,49.12 55.85,45.4 R51.1
TXLED9
  Top 0.203: 69.65,53.21 69.66,53.21 69.66,52.74 70.16,52.24 70.16,51.03 70.47,50.72 70.47,49.94 70.63,49.78 72.62,49.78 72.99,49.41 73.86,49.41 74.14,49.12 74.14,45.4 R57.1
TXLED10
  Top 0.203: 87.94,53.21 87.95,53.21 87.95,52.74 88.44,52.24 88.44,51.03 88.76,50.72 88.76,49.94 88.92,49.78 90.91,49.78 91.28,49.41 92.14,49.41 92.43,49.12 92.43,45.4 R63.1
TXLED11
  Top 0.203: 106.22,53.21 106.23,53.21 106.24,53.21 106.24,52.74 106.73,52.24 106.73,51.03 107.05,50.72 107.05,49.94 107.21,49.78 109.2,49.78 109.56,49.41 110.43,49.41 110.72,49.12 110.72,45.4 R69.1
TXLED12
  Top 0.203: 14.78,90.04 14.79,90.04 14.8,90.04 14.8,89.57 15.29,89.07 15.29,87.86 15.61,87.55 15.61,86.77 15.77,86.61 17.76,86.61 18.12,86.24 18.99,86.24 19.28,85.95 19.28,82.23 R75.1
TXLED13
  Top 0.203: 33.07,90.04 33.08,90.04 33.08,89.57 33.58,89.07 33.58,87.86 33.9,87.55 33.9,86.77 34.06,86.61 36.05,86.61 36.41,86.24 37.28,86.24 37.57,85.95 37.57,82.23 R81.1
TXLED14
  Top 0.203: 51.36,90.04 51.37,90.04 51.37,89.57 51.87,89.07 51.87,87.86 52.18,87.55 52.18,86.77 52.34,86.61 54.33,86.61 54.7,86.24 55.57,86.24 55.85,85.95 55.85,82.23 R87.1
TXLED15
  Top 0.203: 69.65,90.04 69.66,90.04 69.66,89.57 70.16,89.07 70.16,87.86 70.47,87.55 70.47,86.77 70.63,86.61 72.62,86.61 72.99,86.24 73.86,86.24 74.14,85.95 74.14,82.23 R93.1
TXLED16
  Top 0.203: 87.94,90.04 87.95,90.04 87.95,89.57 88.44,89.07 88.44,87.86 88.76,87.55 88.76,86.77 88.92,86.61 90.91,86.61 91.28,86.24 92.14,86.24 92.43,85.95 92.43,82.23 R99.1
TXLED17
  Top 0.203: 106.22,90.04 106.23,90.04 106.24,90.04 106.24,89.57 106.73,89.07 106.73,87.86 107.05,87.55 107.05,86.77 107.21,86.61 109.2,86.61 109.56,86.24 110.43,86.24 110.72,85.95 110.72,82.23 R105.1
TXO  (via drill 0.25)
  Top 0.203: 14.44,16.73 14.4,16.69 14.38,16.69 14.38,15.27 v14.63,15.02
  Bottom 0.203: JP7.12 12.57,31.62 12.53,31.57 12.53,27.91 11.39,26.77 10.78,26.77 10.58,26.58 10.58,24.99 10.65,24.92 11.45,24.92 12.57,23.8 12.57,21.43 15.48,18.52 15.48,15.87 v14.63,15.02
TXO1  (via drill 0.25)
  Top 0.203: 32.72,16.73 32.69,16.69 32.66,16.69 32.66,15.27 v32.92,15.02
  Bottom 0.203: JP4.12 30.86,31.62 30.81,31.57 30.81,27.91 29.68,26.77 29.07,26.77 28.87,26.58 28.87,24.99 28.94,24.92 29.74,24.92 30.86,23.8 30.86,21.43 33.76,18.52 33.76,15.87 v32.92,15.02
TXO2  (via drill 0.25)
  Top 0.203: 51.01,16.73 50.97,16.69 50.95,16.69 50.95,15.27 v51.2,15.02
  Bottom 0.203: JP10.12 49.15,31.62 49.1,31.57 49.1,27.91 47.96,26.77 47.36,26.77 47.16,26.58 47.16,24.99 47.22,24.92 48.02,24.92 49.15,23.8 49.15,21.43 52.05,18.52 52.05,15.87 v51.2,15.02
TXO3  (via drill 0.25)
  Top 0.203: 69.3,16.73 69.26,16.69 69.24,16.69 69.24,15.27 v69.49,15.02
  Bottom 0.203: JP14.12 67.44,31.62 67.39,31.57 67.39,27.91 66.25,26.77 65.64,26.77 65.45,26.58 65.45,24.99 65.51,24.92 66.31,24.92 67.44,23.8 67.44,21.43 70.34,18.52 70.34,15.87 v69.49,15.02
TXO4  (via drill 0.25)
  Top 0.203: 87.59,16.73 87.55,16.69 87.53,16.69 87.53,15.27 v87.78,15.02
  Bottom 0.203: JP18.12 85.72,31.62 85.68,31.57 85.68,27.91 84.54,26.77 83.93,26.77 83.73,26.58 83.73,24.99 83.8,24.92 84.6,24.92 85.72,23.8 85.72,21.43 88.63,18.52 88.63,15.87 v87.78,15.02
TXO5  (via drill 0.25)
  Top 0.203: 105.88,16.73 105.84,16.69 105.82,16.69 105.82,15.27 v106.07,15.02
  Bottom 0.203: JP22.12 104.01,31.62 103.97,31.57 103.97,27.91 102.83,26.77 102.22,26.77 102.02,26.58 102.02,24.99 102.09,24.92 102.89,24.92 104.01,23.8 104.01,21.43 106.92,18.52 106.92,15.87 v106.07,15.02
TXO6  (via drill 0.25)
  Top 0.203: 14.44,53.56 14.4,53.52 14.38,53.52 14.38,52.1 v14.63,51.85
  Bottom 0.203: JP26.12 12.57,68.45 12.53,68.41 12.53,64.74 11.39,63.6 10.78,63.6 10.58,63.41 10.58,61.82 10.65,61.75 11.45,61.75 12.57,60.62 12.57,58.26 15.48,55.35 15.48,52.7 v14.63,51.85
TXO7  (via drill 0.25)
  Top 0.203: 32.72,53.56 32.69,53.52 32.66,53.52 32.66,52.1 v32.92,51.85
  Bottom 0.203: JP30.12 30.86,68.45 30.81,68.41 30.81,64.74 29.68,63.6 29.07,63.6 28.87,63.41 28.87,61.82 28.94,61.75 29.74,61.75 30.86,60.62 30.86,58.26 33.76,55.35 33.76,52.7 v32.92,51.85
TXO8  (via drill 0.25)
  Top 0.203: 51.01,53.56 50.97,53.52 50.95,53.52 50.95,52.1 v51.2,51.85
  Bottom 0.203: JP34.12 49.15,68.45 49.1,68.41 49.1,64.74 47.96,63.6 47.36,63.6 47.16,63.41 47.16,61.82 47.22,61.75 48.02,61.75 49.15,60.62 49.15,58.26 52.05,55.35 52.05,52.7 v51.2,51.85
TXO9  (via drill 0.25)
  Top 0.203: 69.3,53.56 69.26,53.52 69.24,53.52 69.24,52.1 v69.49,51.85
  Bottom 0.203: JP38.12 67.44,68.45 67.39,68.41 67.39,64.74 66.25,63.6 65.64,63.6 65.45,63.41 65.45,61.82 65.51,61.75 66.31,61.75 67.44,60.62 67.44,58.26 70.34,55.35 70.34,52.7 v69.49,51.85
TXO10  (via drill 0.25)
  Top 0.203: 87.59,53.56 87.55,53.52 87.53,53.52 87.53,52.1 v87.78,51.85
  Bottom 0.203: JP42.12 85.72,68.45 85.68,68.41 85.68,64.74 84.54,63.6 83.93,63.6 83.73,63.41 83.73,61.82 83.8,61.75 84.6,61.75 85.72,60.62 85.72,58.26 88.63,55.35 88.63,52.7 v87.78,51.85
TXO11  (via drill 0.25)
  Top 0.203: 105.88,53.56 105.84,53.52 105.82,53.52 105.82,52.1 v106.07,51.85
  Bottom 0.203: JP46.12 104.01,68.45 103.97,68.41 103.97,64.74 102.83,63.6 102.22,63.6 102.02,63.41 102.02,61.82 102.09,61.75 102.89,61.75 104.01,60.62 104.01,58.26 106.92,55.35 106.92,52.7 v106.07,51.85
TXO12  (via drill 0.25)
  Top 0.203: 14.44,90.39 14.4,90.35 14.38,90.35 14.38,88.93 v14.63,88.68
  Bottom 0.203: JP50.12 12.57,105.28 12.53,105.23 12.53,101.57 11.39,100.43 10.78,100.43 10.58,100.24 10.58,98.65 10.65,98.58 11.45,98.58 12.57,97.45 12.57,95.08 15.48,92.18 15.48,89.53 v14.63,88.68
TXO13  (via drill 0.25)
  Top 0.203: 32.72,90.39 32.69,90.35 32.66,90.35 32.66,88.93 v32.92,88.68
  Bottom 0.203: JP54.12 30.86,105.28 30.81,105.23 30.81,101.57 29.68,100.43 29.07,100.43 28.87,100.24 28.87,98.65 28.94,98.58 29.74,98.58 30.86,97.45 30.86,95.08 33.76,92.18 33.76,89.53 v32.92,88.68
TXO14  (via drill 0.25)
  Top 0.203: 51.01,90.39 50.97,90.35 50.95,90.35 50.95,88.93 v51.2,88.68
  Bottom 0.203: JP58.12 49.15,105.28 49.1,105.23 49.1,101.57 47.96,100.43 47.36,100.43 47.16,100.24 47.16,98.65 47.22,98.58 48.02,98.58 49.15,97.45 49.15,95.08 52.05,92.18 52.05,89.53 v51.2,88.68
TXO15  (via drill 0.25)
  Top 0.203: 69.3,90.39 69.26,90.35 69.24,90.35 69.24,88.93 v69.49,88.68
  Bottom 0.203: JP62.12 67.44,105.28 67.39,105.23 67.39,101.57 66.25,100.43 65.64,100.43 65.45,100.24 65.45,98.65 65.51,98.58 66.31,98.58 67.44,97.45 67.44,95.08 70.34,92.18 70.34,89.53 v69.49,88.68
TXO16  (via drill 0.25)
  Top 0.203: 87.59,90.39 87.55,90.35 87.53,90.35 87.53,88.93 v87.78,88.68
  Bottom 0.203: JP66.12 85.72,105.28 85.68,105.23 85.68,101.57 84.54,100.43 83.93,100.43 83.73,100.24 83.73,98.65 83.8,98.58 84.6,98.58 85.72,97.45 85.72,95.08 88.63,92.18 88.63,89.53 v87.78,88.68
TXO17  (via drill 0.25)
  Top 0.203: 105.88,90.39 105.84,90.35 105.82,90.35 105.82,88.93 v106.07,88.68
  Bottom 0.203: JP70.12 104.01,105.28 103.97,105.23 103.97,101.57 102.83,100.43 102.22,100.43 102.02,100.24 102.02,98.65 102.09,98.58 102.89,98.58 104.01,97.45 104.01,95.08 106.92,92.18 106.92,89.53 v106.07,88.68
UVCC  (via drill 0.25)
  Top 0.203: 17.27,31.75 F1.1 17.42,31.89 C6.2 18.71,31.88 18.71,31.18 v18.21,30.68 | v18.92,36.32 18.26,35.66 17.93,35.66 17.78,35.51 17.78,35.18 17.55,34.95 17.14,34.95 17.05,35.05 X1.VBUS1 | v15.87,26.09 14.78,26.09 14.38,25.7 14.38,24.97 14.4,24.97 14.45,24.92 | v11.7,25.98 11.56,25.84 10.21,25.84 9.99,25.63 9.99,24.39 10.21,24.18 11.12,24.18 11.54,23.76 12.15,23.76 12.15,23.73 U3.7
  Bottom 0.203: 18.29,30.76 v18.21,30.68 | v18.21,30.68 18.21,35.61 v18.92,36.32 | v18.21,30.68 18.21,29.56 17.4,28.75 17.4,27.51 15.98,26.09 v15.87,26.09 14.32,27.64 12.8,27.64 11.7,26.54 v11.7,25.98
UVCC1  (via drill 0.25)
  Top 0.203: 35.56,31.75 F2.1 35.7,31.89 C17.2 37,31.88 37,31.18 v36.5,30.68 | v37.21,36.32 36.55,35.66 36.22,35.66 36.07,35.51 36.07,35.18 35.84,34.95 35.43,34.95 35.34,35.05 X2.VBUS1 | v34.16,26.09 33.06,26.09 32.67,25.7 32.67,24.97 32.69,24.97 32.73,24.92 | v29.99,25.98 29.85,25.84 28.5,25.84 28.28,25.63 28.28,24.39 28.49,24.18 29.41,24.18 29.82,23.76 30.44,23.76 30.44,23.73 U4.7
  Bottom 0.203: 36.58,30.76 v36.5,30.68 | v36.5,30.68 36.5,35.61 v37.21,36.32 | v36.5,30.68 36.5,29.56 35.68,28.75 35.68,27.51 34.27,26.09 v34.16,26.09 32.61,27.64 31.09,27.64 29.99,26.54 v29.99,25.98
UVCC2  (via drill 0.25)
  Top 0.203: 53.85,31.75 F3.1 53.99,31.89 C27.2 55.28,31.88 55.28,31.18 v54.79,30.68 | v55.5,36.32 54.84,35.66 54.51,35.66 54.36,35.51 54.36,35.18 54.13,34.95 53.72,34.95 53.62,35.05 X3.VBUS1 | v52.45,26.09 51.35,26.09 50.96,25.7 50.96,24.97 50.98,24.97 51.02,24.92 | v48.27,25.98 48.14,25.84 46.79,25.84 46.57,25.63 46.57,24.39 46.78,24.18 47.7,24.18 48.11,23.76 48.73,23.76 48.73,23.73 U6.7
  Bottom 0.203: 54.86,30.76 v54.79,30.68 | v54.79,30.68 54.79,35.61 v55.5,36.32 | v54.79,30.68 54.79,29.56 53.97,28.75 53.97,27.51 52.55,26.09 v52.45,26.09 50.9,27.64 49.37,27.64 48.27,26.54 v48.27,25.98
UVCC3  (via drill 0.25)
  Top 0.203: 72.14,31.75 F4.1 72.28,31.89 C36.2 73.57,31.18 v73.08,30.68 | v73.79,36.32 73.13,35.66 72.8,35.66 72.64,35.51 72.64,35.18 72.42,34.95 72.01,34.95 71.91,35.05 X4.VBUS1 | v70.73,26.09 69.64,26.09 69.25,25.7 69.25,24.97 69.26,24.97 69.31,24.92 | v66.56,25.98 66.43,25.84 65.08,25.84 64.86,25.63 64.86,24.39 65.07,24.18 65.99,24.18 66.4,23.76 67.01,23.76 67.01,23.73 U8.7
  Bottom 0.203: 73.15,30.76 v73.08,30.68 | v73.08,30.68 73.08,35.61 v73.79,36.32 | v73.08,30.68 73.08,29.56 72.26,28.75 72.26,27.51 70.84,26.09 v70.73,26.09 69.19,27.64 67.66,27.64 66.56,26.54 v66.56,25.98
UVCC4  (via drill 0.25)
  Top 0.203: 90.43,31.75 F5.1 90.57,31.89 C45.2 91.86,31.18 v91.36,30.68 | v92.08,36.32 91.42,35.66 91.08,35.66 90.93,35.51 90.93,35.18 90.7,34.95 90.3,34.95 90.2,35.05 X5.VBUS1 | v89.02,26.09 87.93,26.09 87.53,25.7 87.53,24.97 87.55,24.97 87.6,24.92 | v84.85,25.98 84.71,25.84 83.36,25.84 83.15,25.63 83.15,24.39 83.36,24.18 84.28,24.18 84.69,23.76 85.3,23.76 85.3,23.73 U10.7
  Bottom 0.203: 91.44,30.76 v91.36,30.68 | v91.36,30.68 91.36,35.61 v92.08,36.32 | v91.36,30.68 91.36,29.56 90.55,28.75 90.55,27.51 89.13,26.09 v89.02,26.09 87.47,27.64 85.95,27.64 84.85,26.54 v84.85,25.98
UVCC5  (via drill 0.25)
  Top 0.203: 108.72,31.75 F6.1 108.86,31.89 C54.2 110.15,31.88 110.15,31.18 v109.65,30.68 | v110.36,36.32 109.7,35.66 109.37,35.66 109.22,35.51 109.22,35.18 108.99,34.95 108.58,34.95 108.49,35.05 X6.VBUS1 | v107.31,26.09 106.22,26.09 105.82,25.7 105.82,24.97 105.84,24.97 105.89,24.92 | v103.14,25.98 103,25.84 101.65,25.84 101.44,25.63 101.44,24.39 101.65,24.18 102.56,24.18 102.98,23.76 103.59,23.76 103.59,23.73 U12.7
  Bottom 0.203: 109.73,30.76 v109.65,30.68 | v109.65,30.68 109.65,35.61 v110.36,36.32 | v109.65,30.68 109.65,29.56 108.84,28.75 108.84,27.51 107.42,26.09 v107.31,26.09 105.76,27.64 104.24,27.64 103.14,26.54 v103.14,25.98
UVCC6  (via drill 0.25)
  Top 0.203: 17.27,68.58 F7.1 17.42,68.72 C63.2 18.71,68.71 18.71,68.01 v18.21,67.51 | v18.92,73.15 18.26,72.49 17.93,72.49 17.78,72.34 17.78,72.01 17.55,71.78 17.14,71.78 17.05,71.88 X7.VBUS1 | v15.87,62.92 14.78,62.92 14.38,62.53 14.38,61.8 14.4,61.8 14.45,61.75 | v11.7,62.81 11.56,62.67 10.21,62.67 9.99,62.46 9.99,61.22 10.21,61.01 11.12,61.01 11.54,60.59 12.15,60.59 12.15,60.56 U14.7
  Bottom 0.203: 18.29,67.59 v18.21,67.51 | v18.21,67.51 18.21,72.44 v18.92,73.15 | v18.21,67.51 18.21,66.39 17.4,65.58 17.4,64.34 15.98,62.92 v15.87,62.92 14.32,64.47 12.8,64.47 11.7,63.37 v11.7,62.81
UVCC7  (via drill 0.25)
  Top 0.203: 35.56,68.58 F8.1 35.7,68.72 C72.2 37,68.71 37,68.01 v36.5,67.51 | v37.21,73.15 36.55,72.49 36.22,72.49 36.07,72.34 36.07,72.01 35.84,71.78 35.43,71.78 35.34,71.88 X8.VBUS1 | v34.16,62.92 33.06,62.92 32.67,62.53 32.67,61.8 32.69,61.8 32.73,61.75 | v29.99,62.81 29.85,62.67 28.5,62.67 28.28,62.46 28.28,61.22 28.49,61.01 29.41,61.01 29.82,60.59 30.44,60.59 30.44,60.56 U16.7
  Bottom 0.203: 36.58,67.59 v36.5,67.51 | v36.5,67.51 36.5,72.44 v37.21,73.15 | v36.5,67.51 36.5,66.39 35.68,65.58 35.68,64.34 34.27,62.92 v34.16,62.92 32.61,64.47 31.09,64.47 29.99,63.37 v29.99,62.81
UVCC8  (via drill 0.25)
  Top 0.203: 53.85,68.58 F9.1 53.99,68.72 C81.2 55.28,68.71 55.28,68.01 v54.79,67.51 | v55.5,73.15 54.84,72.49 54.51,72.49 54.36,72.34 54.36,72.01 54.13,71.78 53.72,71.78 53.62,71.88 X9.VBUS1 | v52.45,62.92 51.35,62.92 50.96,62.53 50.96,61.8 50.98,61.8 51.02,61.75 | v48.27,62.81 48.14,62.67 46.79,62.67 46.57,62.46 46.57,61.22 46.78,61.01 47.7,61.01 48.11,60.59 48.73,60.59 48.73,60.56 U18.7
  Bottom 0.203: 54.86,67.59 v54.79,67.51 | v54.79,67.51 54.79,72.44 v55.5,73.15 | v54.79,67.51 54.79,66.39 53.97,65.58 53.97,64.34 52.55,62.92 v52.45,62.92 50.9,64.47 49.37,64.47 48.27,63.37 v48.27,62.81
UVCC9  (via drill 0.25)
  Top 0.203: 72.14,68.58 F10.1 72.28,68.72 C90.2 73.57,68.01 v73.08,67.51 | v73.79,73.15 73.13,72.49 72.8,72.49 72.64,72.34 72.64,72.01 72.42,71.78 72.01,71.78 71.91,71.88 X10.VBUS1 | v70.73,62.92 69.64,62.92 69.25,62.53 69.25,61.8 69.26,61.8 69.31,61.75 | v66.56,62.81 66.43,62.67 65.08,62.67 64.86,62.46 64.86,61.22 65.07,61.01 65.99,61.01 66.4,60.59 67.01,60.59 67.01,60.56 U20.7
  Bottom 0.203: 73.15,67.59 v73.08,67.51 | v73.08,67.51 73.08,72.44 v73.79,73.15 | v73.08,67.51 73.08,66.39 72.26,65.58 72.26,64.34 70.84,62.92 v70.73,62.92 69.19,64.47 67.66,64.47 66.56,63.37 v66.56,62.81
UVCC10  (via drill 0.25)
  Top 0.203: 90.43,68.58 F11.1 90.57,68.72 C99.2 91.86,68.01 v91.36,67.51 | v92.08,73.15 91.42,72.49 91.08,72.49 90.93,72.34 90.93,72.01 90.7,71.78 90.3,71.78 90.2,71.88 X11.VBUS1 | v89.02,62.92 87.93,62.92 87.53,62.53 87.53,61.8 87.55,61.8 87.6,61.75 | v84.85,62.81 84.71,62.67 83.36,62.67 83.15,62.46 83.15,61.22 83.36,61.01 84.28,61.01 84.69,60.59 85.3,60.59 85.3,60.56 U22.7
  Bottom 0.203: 91.44,67.59 v91.36,67.51 | v91.36,67.51 91.36,72.44 v92.08,73.15 | v91.36,67.51 91.36,66.39 90.55,65.58 90.55,64.34 89.13,62.92 v89.02,62.92 87.47,64.47 85.95,64.47 84.85,63.37 v84.85,62.81
UVCC11  (via drill 0.25)
  Top 0.203: 108.72,68.58 F12.1 108.86,68.72 C108.2 110.15,68.71 110.15,68.01 v109.65,67.51 | v110.36,73.15 109.7,72.49 109.37,72.49 109.22,72.34 109.22,72.01 108.99,71.78 108.58,71.78 108.49,71.88 X12.VBUS1 | v107.31,62.92 106.22,62.92 105.82,62.53 105.82,61.8 105.84,61.8 105.89,61.75 | v103.14,62.81 103,62.67 101.65,62.67 101.44,62.46 101.44,61.22 101.65,61.01 102.56,61.01 102.98,60.59 103.59,60.59 103.59,60.56 U24.7
  Bottom 0.203: 109.73,67.59 v109.65,67.51 | v109.65,67.51 109.65,72.44 v110.36,73.15 | v109.65,67.51 109.65,66.39 108.84,65.58 108.84,64.34 107.42,62.92 v107.31,62.92 105.76,64.47 104.24,64.47 103.14,63.37 v103.14,62.81
UVCC12  (via drill 0.25)
  Top 0.203: 17.27,105.41 F13.1 17.42,105.55 C117.2 18.71,105.54 18.71,104.84 v18.21,104.34 | v18.92,109.98 18.26,109.32 17.93,109.32 17.78,109.17 17.78,108.84 17.55,108.61 17.14,108.61 17.05,108.71 X13.VBUS1 | v15.87,99.75 14.78,99.75 14.38,99.36 14.38,98.63 14.4,98.63 14.45,98.58 | v11.7,99.64 11.56,99.5 10.21,99.5 9.99,99.29 9.99,98.05 10.21,97.84 11.12,97.84 11.54,97.42 12.15,97.42 12.15,97.39 U26.7
  Bottom 0.203: 18.29,104.42 v18.21,104.34 | v18.21,104.34 18.21,109.27 v18.92,109.98 | v18.21,104.34 18.21,103.22 17.4,102.41 17.4,101.17 15.98,99.75 v15.87,99.75 14.32,101.3 12.8,101.3 11.7,100.2 v11.7,99.64
UVCC13  (via drill 0.25)
  Top 0.203: 35.56,105.41 F14.1 35.7,105.55 C126.2 37,105.54 37,104.84 v36.5,104.34 | v37.21,109.98 36.55,109.32 36.22,109.32 36.07,109.17 36.07,108.84 35.84,108.61 35.43,108.61 35.34,108.71 X14.VBUS1 | v34.16,99.75 33.06,99.75 32.67,99.36 32.67,98.63 32.69,98.63 32.73,98.58 | v29.99,99.64 29.85,99.5 28.5,99.5 28.28,99.29 28.28,98.05 28.49,97.84 29.41,97.84 29.82,97.42 30.44,97.42 30.44,97.39 U28.7
  Bottom 0.203: 36.58,104.42 v36.5,104.34 | v36.5,104.34 36.5,109.27 v37.21,109.98 | v36.5,104.34 36.5,103.22 35.68,102.41 35.68,101.17 34.27,99.75 v34.16,99.75 32.61,101.3 31.09,101.3 29.99,100.2 v29.99,99.64
UVCC14  (via drill 0.25)
  Top 0.203: 53.85,105.41 F15.1 53.99,105.55 C135.2 55.28,105.54 55.28,104.84 v54.79,104.34 | v55.5,109.98 54.84,109.32 54.51,109.32 54.36,109.17 54.36,108.84 54.13,108.61 53.72,108.61 53.62,108.71 X15.VBUS1 | v52.45,99.75 51.35,99.75 50.96,99.36 50.96,98.63 50.98,98.63 51.02,98.58 | v48.27,99.64 48.14,99.5 46.79,99.5 46.57,99.29 46.57,98.05 46.78,97.84 47.7,97.84 48.11,97.42 48.73,97.42 48.73,97.39 U30.7
  Bottom 0.203: 54.86,104.42 v54.79,104.34 | v54.79,104.34 54.79,109.27 v55.5,109.98 | v54.79,104.34 54.79,103.22 53.97,102.41 53.97,101.17 52.55,99.75 v52.45,99.75 50.9,101.3 49.37,101.3 48.27,100.2 v48.27,99.64
UVCC15  (via drill 0.25)
  Top 0.203: 72.14,105.41 F16.1 72.28,105.55 C144.2 73.57,104.84 v73.08,104.34 | v73.79,109.98 73.13,109.32 72.8,109.32 72.64,109.17 72.64,108.84 72.42,108.61 72.01,108.61 71.91,108.71 X16.VBUS1 | v70.73,99.75 69.64,99.75 69.25,99.36 69.25,98.63 69.26,98.63 69.31,98.58 | v66.56,99.64 66.43,99.5 65.08,99.5 64.86,99.29 64.86,98.05 65.07,97.84 65.99,97.84 66.4,97.42 67.01,97.42 67.01,97.39 U32.7
  Bottom 0.203: 73.15,104.42 v73.08,104.34 | v73.08,104.34 73.08,109.27 v73.79,109.98 | v73.08,104.34 73.08,103.22 72.26,102.41 72.26,101.17 70.84,99.75 v70.73,99.75 69.19,101.3 67.66,101.3 66.56,100.2 v66.56,99.64
UVCC16  (via drill 0.25)
  Top 0.203: 90.43,105.41 F17.1 90.57,105.55 C153.2 91.86,104.84 v91.36,104.34 | v92.08,109.98 91.42,109.32 91.08,109.32 90.93,109.17 90.93,108.84 90.7,108.61 90.3,108.61 90.2,108.71 X17.VBUS1 | v89.02,99.75 87.93,99.75 87.53,99.36 87.53,98.63 87.55,98.63 87.6,98.58 | v84.85,99.64 84.71,99.5 83.36,99.5 83.15,99.29 83.15,98.05 83.36,97.84 84.28,97.84 84.69,97.42 85.3,97.42 85.3,97.39 U34.7
  Bottom 0.203: 91.44,104.42 v91.36,104.34 | v91.36,104.34 91.36,109.27 v92.08,109.98 | v91.36,104.34 91.36,103.22 90.55,102.41 90.55,101.17 89.13,99.75 v89.02,99.75 87.47,101.3 85.95,101.3 84.85,100.2 v84.85,99.64
UVCC17  (via drill 0.25)
  Top 0.203: 108.72,105.41 F18.1 108.86,105.55 C162.2 110.15,105.54 110.15,104.84 v109.65,104.34 | v110.36,109.98 109.7,109.32 109.37,109.32 109.22,109.17 109.22,108.84 108.99,108.61 108.58,108.61 108.49,108.71 X18.VBUS1 | v107.31,99.75 106.22,99.75 105.82,99.36 105.82,98.63 105.84,98.63 105.89,98.58 | v103.14,99.64 103,99.5 101.65,99.5 101.44,99.29 101.44,98.05 101.65,97.84 102.56,97.84 102.98,97.42 103.59,97.42 103.59,97.39 U36.7
  Bottom 0.203: 109.73,104.42 v109.65,104.34 | v109.65,104.34 109.65,109.27 v110.36,109.98 | v109.65,104.34 109.65,103.22 108.84,102.41 108.84,101.17 107.42,99.75 v107.31,99.75 105.76,101.3 104.24,101.3 103.14,100.2 v103.14,99.64
VCC  (via drill 0.25)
